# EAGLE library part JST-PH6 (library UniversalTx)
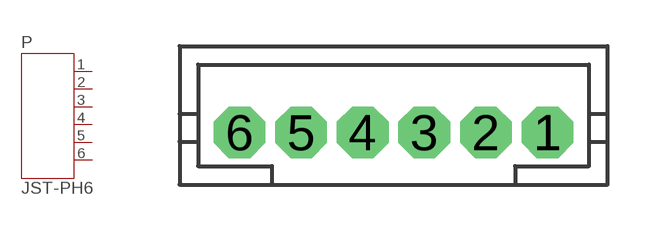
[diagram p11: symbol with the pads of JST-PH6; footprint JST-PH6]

Designator prefix P

## JST-PH6  [JST-PH6]
1  1  pas
2  2  pas
3  3  pas
4  4  pas
5  5  pas
6  6  pas

## Footprint JST-PH6 (pad centres in mm)
drill 0.813 pad 1.676 octagon: 1 5,0; 2 3,0; 3 1,0; 4 -1,0; 5 -3,0; 6 -5,0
